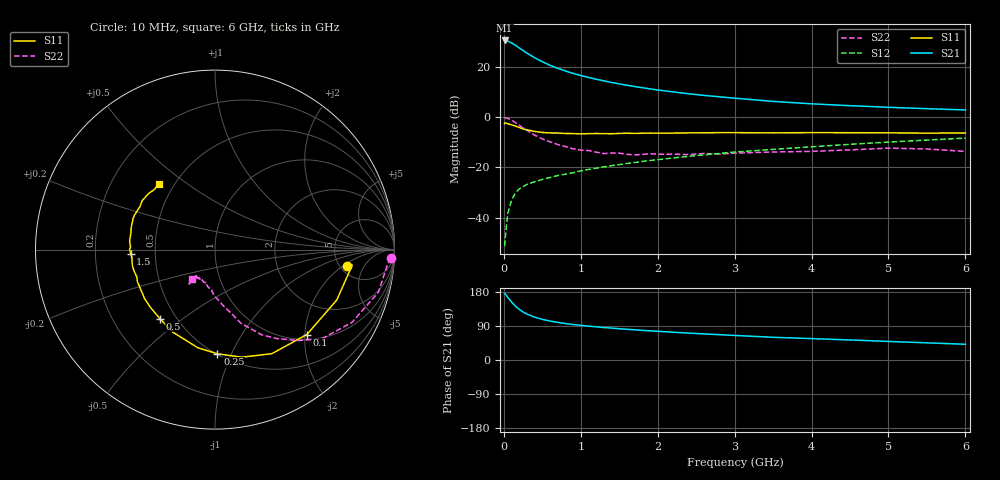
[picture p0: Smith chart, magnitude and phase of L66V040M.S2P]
!  INFINEON TECHNOLOGIES Small Signal Semiconductors
! BFR380L3 , Si-NPN RF-Transistor in TSLP-3-1
!  Vce=6 V,  Ic=40 mA
! Common Emitter S-Parameters:  07. March 2005
#  GHz  S  MA  R  50
! f  S11  S21  S12  S22
! GHz  Mag  Ang  Mag  Ang  Mag  Ang  Mag  Ang
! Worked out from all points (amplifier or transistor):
!   36 points, 10 MHz to 6 GHz, reference 50 ohm
!   highest |S21| = 30.4 dB at 10 MHz (marker M1)
!   |S21| within 3 dB of that: start of sweep to 202.2 MHz
!   unconditionally stable (mu >= 1): 1.937 GHz to 4.795 GHz
!   at 250 MHz: K = 0.38, MSG = 27.1 dB, |S12| = -27.7 dB
!   at 1.4 GHz: K = 0.95, MSG = 16.6 dB, |S12| = -19.4 dB
!   at 6 GHz: K = 0.97, MSG = 5.6 dB, |S12| = -8.4 dB
!   S11 on the Smith chart (normalised r, x): 10 MHz: 5.77, -2.26; 100 MHz: 1.11, -2.05; 250 MHz: 0.51, -0.89; 500 MHz: 0.41, -0.41; 1.5 GHz: 0.36, -0.02; 6 GHz: 0.41, +0.40
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0.01  0.7394 -6.9  33.2 175.0  0.0027 73.5  0.9793 -2.7
0.02  0.7698 -6.4  33.2 174.2  0.0041 81.2  0.9609 -5.9
0.05  0.7341 -22.5  32.2 165.6  0.0119 79.5  0.9406 -14.7
0.1  0.6971 -42.8  29.65 153.0  0.0224 70.5  0.8641 -28.0
0.15  0.6608 -61.4  26.71 142.1  0.0307 62.9  0.7761 -39.7
0.2  0.6171 -76.2  23.63 133.5  0.037 60.0  0.6868 -47.6
0.25  0.5805 -88.7  20.96 126.9  0.041 55.4  0.6024 -55.3
0.3  0.5554 -99.8  18.59 121.2  0.0457 55.1  0.5423 -61.2
0.4  0.517 -116.6  15.09 113.0  0.0516 53.8  0.4352 -70.6
0.5  0.4923 -128.7  12.55 107.3  0.0573 53.5  0.3669 -75.6
0.6  0.4827 -138.2  10.65 102.8  0.0624 54.6  0.321 -81.0
0.7  0.478 -145.1  9.293 99.3  0.0683 55.9  0.2839 -85.9
0.9  0.4678 -157.7  7.347 93.7  0.0779 58.2  0.2325 -94.2
1.1  0.4664 -165.0  6.1 89.4  0.0905 60.0  0.2152 -99.6
1.5  0.4702 -177.3  4.544 82.4  0.1129 62.2  0.191 -109.5
1.8  0.4753 175.9  3.814 78.2  0.1306 63.5  0.1796 -115.0
2.2  0.4778 168.6  3.15 73.3  0.1532 64.0  0.1822 -119.0
2.8  0.4884 159.0  2.514 66.8  0.188 64.4  0.1834 -126.6
3.5  0.4821 149.9  2.042 59.9  0.2268 62.9  0.2012 -126.5
4.5  0.4865 143.6  1.676 52.9  0.286 61.8  0.2215 -126.9
5.5  0.4761 135.5  1.461 45.3  0.3473 58.6  0.2311 -126.7
6  0.482 130.2  1.381 41.5  0.38 56.6  0.2065 -127.6
